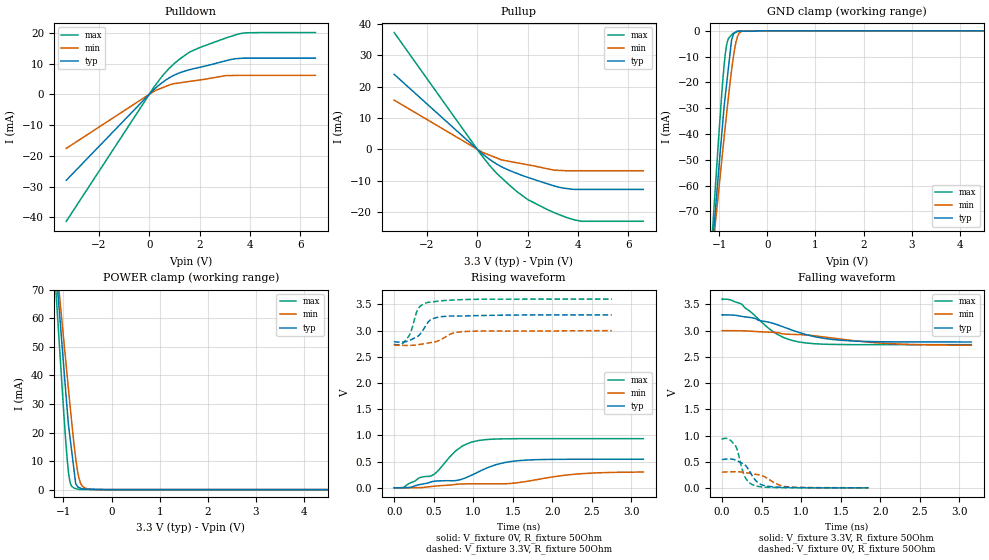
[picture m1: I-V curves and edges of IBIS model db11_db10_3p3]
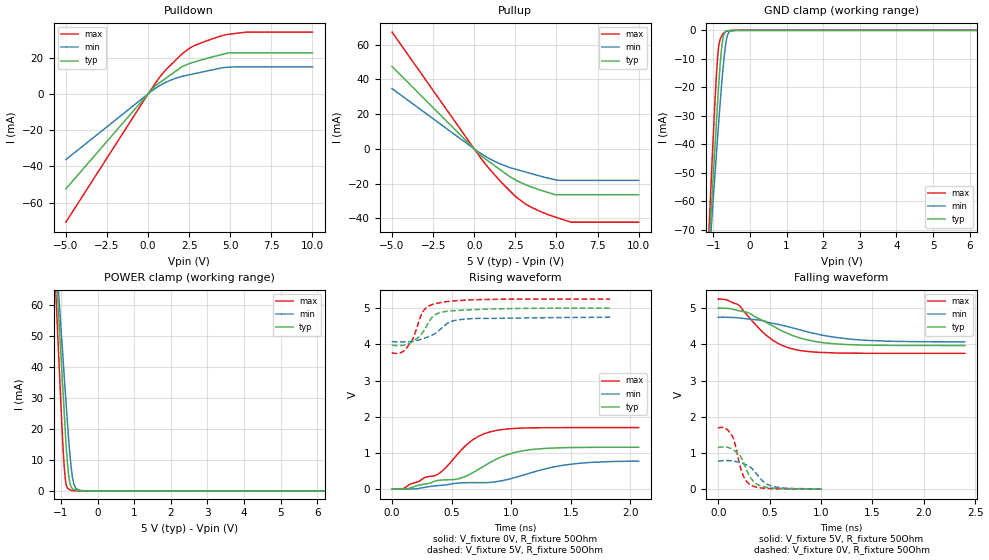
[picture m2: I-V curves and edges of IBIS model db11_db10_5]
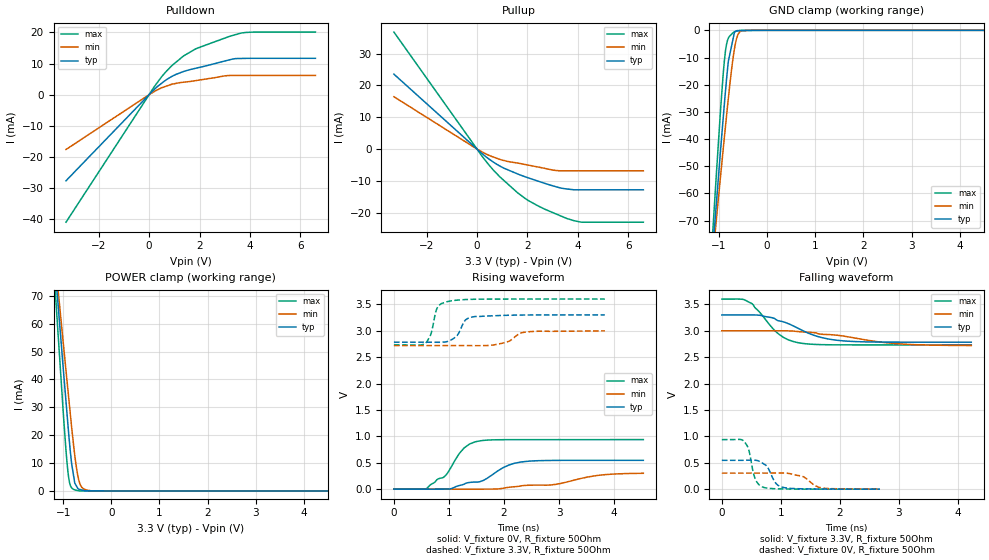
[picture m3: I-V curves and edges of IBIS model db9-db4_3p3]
|Texas Instruments Incorporated
| 2.7V-5.25V Digital, 5V Analog, 12 Bit, 3MSPS, Parallel ADC with Ref
| Marketing part#   Digital Voltage Range   Package-type   #pins
| ADS7882IPFBR   2.7V-5.25V   TQFP   48
| ADS7882IPFBT   2.7V-5.25V   TQFP   48
[IBIS Ver]   3.2
[File name]   ads7882.ibs
|SIMDE Ver   V2.2 - 201009 - RHL4 - Build 424
[File Rev]   1.1
[Date]   4/15/2011
[Source]
| Texas Instruments Incorporated.
| Analog-eLab Design Center, HPA
| 12500 TI Blvd
| Dallas, TX -75243
| e-mail: elab_ibis@list.ti.com
| -Model generated from simulations in SPECTRE
[Notes]   Revision History:
| Rev 1.0: 4/8/2011
| - Initial version of the model
| - Model generated from simulations in SPECTRE
| - Model matched to SPICE simulation
| - C_comp although listed in numerical order of value are
|   obtained from varying PVT conditions. For PVT conditions for
|   each specific value refer the buffer description under
|   respective [Model]. IBIS model user is responsible for using
|   appropriate C_comp to simulate for Signal Integrity.
| - Model names with a trailing _3p3 contains the model for
|   3.3V [3.0V and 3.6V].Model names with a trailing _5 contains
|   the model for 5.0V [4.75V and 5.25V].
|   Rev 1.1: 4/15/2011
| - Updated the IBIS model with LC tank C_Comp
[Disclaimer]
| This model is designed as an aid for customers of Texas Instruments.
| TI and its licensors and suppliers make no warranties, either expressed
| or implied, with respect to this  model, including the warranties of
| merchantability or fitness for a particular purpose. The model is
| provided solely on an "as is" basis. The entire risk as to its quality
| and performance is with the customer.
[Copyright]
 (C) Copyright 2011 Texas Instruments Incorporated.All rights reserved.
|   ADS7882
[Component]   ADS7882
[Manufacturer]   TI
[Package]   |48 TQFP - PFB package
|   typ   min   max
R_pkg   0.096154   0.08201   0.10924
L_pkg   2.99219nH   2.49975nH   3.83153nH
C_pkg   0.482595pF   0.40017pF   0.58535pF
[Pin]  signal_name   model_name   R_pin   L_pin   C_pin
1   REFIN   TERM   0.10156   3.67689nH  0.57752pF
2   REFOUT   TERM   0.09278   2.95431nH  0.50865pF
3   NC   NC   0.08775   2.81037nH  0.48710pF
4   +VA   POWER   0.08458   2.75529nH  0.48008pF
5   AGND   GND   0.08266   2.53910nH  0.43335pF
6   IN+   TERM   0.08227   2.50412nH  0.40022pF
7   -IN   TERM   0.08210   2.49975nH  0.40017pF
8   AGND   GND   0.08205   2.52717nH  0.43280pF
9   +VA   POWER   0.08351   2.73719nH  0.47819pF
10   +VA   POWER   0.08625   2.78317nH  0.48546pF
11   AGND   GND   0.09077   2.91560nH  0.51015pF
12   AGND   GND   0.04966   3.05669nH  0.63306pF
13   +VA   POWER   0.11087   3.87375nH  0.58548pF
14   AGND   GND   0.10407   3.18780nH  0.51804pF
15   AGND   GND   0.10062   3.07419nH  0.49891pF
16   DB11   DB   0.09878   3.04135nH  0.49726pF
17   DB10   DB   0.09794   2.84794nH  0.45076pF
18   DB9   DB9-DB3   0.09833   2.82757nH  0.41819pF
19   DB8   DB9-DB3   0.09865   2.83183nH  0.41907pF
20   DB7   DB9-DB3   0.09892   2.86570nH  0.45238pF
21   DB6   DB9-DB3   0.10045   3.07454nH  0.49862pF
22   DB5   DB9-DB3   0.10298   3.12010nH  0.50228pF
23   DB4   DB9-DB3   0.10708   3.24374nH  0.52526pF
24   +VBD   POWER   0.11463   3.93871nH  0.59461pF
25   BDGND   GND   0.09909   3.63469nH  0.57452pF
26   DB3   DB9-DB3   0.09081   2.92111nH  0.50606pF
27   DB2   DB   0.08620   2.78437nH  0.48513pF
28   DB1   DB   0.08347   2.73669nH  0.47871pF
29   DB0   DB0   0.08201   2.52810nH  0.43255pF
30   NC   NC   0.08207   2.50072nH  0.39994pF
31   NC   NC   0.08234   2.50365nH  0.40065pF
32   NC   NC   0.08284   2.54077nH  0.43406pF
33   NC   NC   0.08487   2.76069nH  0.47992pF
34   +VBD   POWER   0.08812   2.81537nH  0.48776pF
35   BDGND   GND   0.09307   2.95530nH  0.51266pF
36   BUSY   BUSY   0.10188   3.67198nH  0.58535pF
37   _A_PWD   INPUT   0.10924   3.83153nH  0.58324pF
38   _PWD/_RST   INPUT   0.10264   3.15016nH  0.51710pF
39   BYTE   BYTE   0.09952   3.04261nH  0.49838pF
40   _CONVST   INPUT   0.09803   3.01798nH  0.49502pF
41   _RD   INPUT   0.09757   2.83036nH  0.44993pF
42   _CS   INPUT   0.09834   2.81763nH  0.41784pF
43   +VA   POWER   0.09896   2.82837nH  0.41883pF
44   AGND   GND   0.09951   2.86775nH  0.45275pF
45   AGND   GND   0.10137   3.08409nH  0.49933pF
46   +VA   POWER   0.10424   3.13488nH  0.50621pF
47   REFM   GND   0.05396   2.70861nH  0.58111pF
48   REFM   GND   0.10969   3.82962nH  0.59256pF
|   Model Selectors
[Model Selector] DB
db11_db10_3p3   3.3V digital 3-state output
db11_db10_5   5.0V digital 3-state output
[Model Selector] DB9-DB3
db9-db4_3p3   3.3V digital 3-state output
db9-db4_5   5.0V digital 3-state output
[Model Selector] DB0
db0_par_3p3   3.3V digital 3-state output
db0_par_5   5.0V digital 3-state output
[Model Selector] BUSY
busy_3p3   3.3V digital output
busy_5   5.0V digital output
[Model Selector] INPUT
input_3p3   3.3V digital input
input_5   5.0V digital input
[Model Selector] BYTE
byte_3p3   3.3V digital input
byte_5   5.0V digital input
[Model Selector] TERM
term_3-3V   3.3V nominal termination
term_5-0V   5.0V nominal termination
[Model]  term_3-3V
Model_type Terminator
C_comp   1.0e-20F  1.0e-20F  1.0e-20F
|   typ   min   max
[Voltage Range]   3.3V   3.0V   3.6V
[POWER Clamp Reference]   3.3V   3.0V   3.6V
[GND Clamp Reference]   0V   0V   0V
|Ambient Temperature   25   85   -40
|Junction Temperature
[Temperature Range]   25   85   -40
[Model]  term_5-0V
Model_type Terminator
C_comp   1.0e-20F  1.0e-20F  1.0e-20F
|   typ   min   max
[Voltage Range]   5.0V   4.75V   5.25V
[POWER Clamp Reference]   5.0V   4.75V   5.25V
[GND Clamp Reference]   0V   0V   0V
|Ambient Temperature   25   85   -40
|Junction Temperature
[Temperature Range]   25   85   -40
| Models and submodels in the file (14): db11_db10_3p3 (3-state), db11_db10_5 (3-state), db9-db4_3p3 (3-state), db9-db4_5 (3-state), db0_par_3p3 (3-state), db0_par_5 (3-state), busy_3p3 (Output), busy_5 (Output), input_3p3 (Input), input_5 (Input), byte_3p3 (Input), byte_5 (Input), term_3-3V (Terminator), term_5-0V (Terminator)
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|   db11_db10_3p3 Model
[Model]   db11_db10_3p3
Model_type   3-state
Polarity   Non-Inverting
Enable   Active-Low
Vmeas = 1.65
Vref = 1.65
Cref = 20pF
Rref = 50
|   typ   min   max
|   (nom PVT)   (Fast PVT)   (slow PVT)
|C_comp from frequency sweep method (F=1.5MHz)
|Average
C_comp   1.207e-12   1.083e-12   1.350e-12
|ON state : BUFFER OUTPUT TURNED HIGH
|C_comp   1.164e-12   1.043e-12   1.312e-12
|OFF state: BUFFER IN HIGH IMPEDANCE
|C_comp   1.251e-12   1.124e-12   1.388e-12
|C_comp from LC tank measurement(L=1nH)
|Resonant Frequency(Hz)   5.950e+09   6.040e+09   5.790e+09
|C_comp   7.162e-13   6.950e-13   7.564e-13
|ON state : BUFFER OUTPUT TURNED HIGH
|Resonant Frequency(Hz)   5.950e+09   6.040e+09   5.790e+09
|C_comp   7.162e-13   6.950e-13   7.564e-13
|OFF state: BUFFER IN HIGH IMPEDANCE
|Resonant Frequency   5.980e+09   6.040e+09   5.270e+09
|C_comp   7.091e-13   6.950e-13   9.130e-13
| Where nom  PVT is Nominal Process,  3.3V,  25C
|   Fast PVT is Strong Process,   3.6V,  -40C
|   Slow PVT is Weak Process,   3V,  85C
[Voltage Range]   3.3   3   3.6
|Ambient Temperature   25   85   -40
|Junction Temperature
[Temperature Range]   25   85   -40
[Pullup Reference]   3.3   3   3.6
[Pulldown Reference]   0   0   0
[Power Clamp Reference]   3.3   3   3.6
[GND Clamp Reference]   0   0   0
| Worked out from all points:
|   slope of the pulldown table from 0 to 0.495 V, typ, clamps not added: 134 ohm
|   slope of the pullup table from 0 to 0.495 V, typ, clamps not added: 152 ohm
|   GND clamp passes 1 mA (typ) near -0.69 V on its own axis
|   POWER clamp passes 1 mA (typ) near -0.70 V on its own axis
|   falling waveform, V_fixture 3.3V, R_fixture 50Ohm: 20-80 % time 702ps typ, 1.13ns min, 431ps max; typ from 3.3 V to 2.78 V
|   rising waveform, V_fixture 0V, R_fixture 50Ohm: 20-80 % time 821ps typ, 1.41ns min, 506ps max; typ from 0 V to 0.545 V
|   rising waveform, V_fixture 3.3V, R_fixture 50Ohm: 20-80 % time 161ps typ, 254ps min, 118ps max; typ from 2.78 V to 3.3 V
|   falling waveform, V_fixture 0V, R_fixture 50Ohm: 20-80 % time 154ps typ, 224ps min, 112ps max; typ from 0.546 V to 0.001 V
[Pulldown]
|   Voltage   I(typ)   I(min)   I(max)
-3.3V     -27.98mA   -17.6mA    -41.31mA
165.6mV   1.385mA    845.6uA    2.114mA
489.6mV   3.669mA    2.022mA    5.683mA
795.6mV   5.364mA    3.005mA    8.487mA
1.256V    7.123mA    3.771mA    11.75mA
1.62V     8.032mA    4.204mA    13.79mA
2.023V    8.799mA    4.669mA    15.25mA
3.024V    10.86mA    6.055mA    18.24mA
3.561V    11.65mA    6.146mA    19.63mA
3.863V    11.74mA    6.146mA    19.99mA
4.392V    11.74mA    6.146mA    20.06mA
6.6V      11.74mA    6.146mA    20.06mA
[GND Clamp]
|   Voltage   I(typ)   I(min)   I(max)
-3.3V     -576.2mA   -485.3mA   -699.8mA
-1.145V   -84.01mA   -86.27mA   -78.64mA
-1.116V   -77.47mA   -80.95mA   -70.35mA
-1.015V   -54.79mA   -62.53mA   -42.05mA
-943.2mV  -38.9mA    -49.37mA   -23.1mA
-874.8mV  -25.19mA   -37.02mA   -8.97mA
-831.6mV  -18.02mA   -29.41mA   -4.204mA
-745.8mV  -3.777mA   -15.46mA   -1.608mA
-640.2mV  -175.5uA   -3.504mA   -449.1uA
-585mV    -160.3uA   -878.4uA   -96.21uA
-441mV    -120.6uA   -12.32uA   -49.56uA
6.6V      0A         0A         0A
[Pullup]
|   Voltage   I(typ)   I(min)   I(max)
-3.3V     23.88mA    15.66mA    37.21mA
133.2mV   -958.5uA   -613uA     -1.531mA
489.6mV   -3.219mA   -1.877mA   -5.159mA
795.6mV   -4.826mA   -2.854mA   -7.853mA
963mV     -5.573mA   -3.388mA   -9.095mA
1.562V    -7.652mA   -4.286mA   -13.42mA
2.023V    -9.002mA   -4.966mA   -16.1mA
2.79V     -11.02mA   -6.217mA   -19.25mA
3.251V    -12.11mA   -6.733mA   -20.84mA
3.863V    -12.8mA    -6.845mA   -22.52mA
4.14V     -12.8mA    -6.845mA   -22.97mA
6.6V      -12.8mA    -6.845mA   -22.97mA
[POWER Clamp]
|   Voltage   I(typ)   I(min)   I(max)
-3.3V     535.6mA    459.6mA    634.1mA
-1.494V   149.6mA    140.6mA    158mA
-1.066V   58.37mA    65.16mA    45.83mA
-954mV    34.64mA    45.45mA    17.39mA
-896.4mV  22.77mA    35.3mA     6.276mA
-849.6mV  16.36mA    27.25mA    1.888mA
-774mV    6.003mA    15.03mA    480.7uA
-742.5mV  1.995mA    10.65mA    356.5uA
-702mV    960.8uA    6.073mA    196.8uA
-642mV    473.3uA    2.131mA    25.18uA
-441mV    169.7uA    94.34uA    10.88uA
6.6V      0A         0A         0A
[Ramp]
R_load = 50
|   typ   min   max
dV/dt_r   0.32766/8.22315e-10   0.182251/1.42229e-09   0.563074/5.05939e-10
dV/dt_f   0.310142/7.04688e-10   0.168714/1.14884e-09   0.520813/4.31957e-10
[Falling Waveform]
V_fixture = 3.3V
V_fixture_min = 3V
V_fixture_max = 3.6V
R_fixture = 50Ohm
|   Time   V(typ)   V(min)   V(max)
0s        3.3V       3V         3.6V
101.4ps   3.299V     3.001V     3.59V
249.2ps   3.272V     2.997V     3.503V
629.5ps   3.147V     2.969V     2.998V
776ps     3.071V     2.939V     2.871V
966.7ps   2.969V     2.925V     2.786V
1.296ns   2.852V     2.879V     2.742V
1.596ns   2.808V     2.822V     2.735V
2.254ns   2.786V     2.744V     2.733V
3.154ns   2.784V     2.722V     2.733V
[Rising Waveform]
V_fixture = 0V
V_fixture_min = 0V
V_fixture_max = 0V
R_fixture = 50Ohm
|   Time   V(typ)   V(min)   V(max)
0s        1.565nV    6.201nV    1.48nV
119.2ps   1.329mV    -140.3uV   11.04mV
317.5ps   60.29mV    3.418mV    190.2mV
484.1ps   119.7mV    27mV       238.9mV
776ps     138.5mV    64.82mV    702mV
1.066ns   304.4mV    76.04mV    902.4mV
1.296ns   444.9mV    76.28mV    931.1mV
1.596ns   521.2mV    104.6mV    937.4mV
2.354ns   544.9mV    267.8mV    937.7mV
3.154ns   545.3mV    301mV      937.9mV
[Rising Waveform]
V_fixture = 3.3V
V_fixture_min = 3V
V_fixture_max = 3.6V
R_fixture = 50Ohm
|   Time   V(typ)   V(min)   V(max)
0s        2.783V     2.719V     2.732V
101.4ps   2.78V      2.717V     2.749V
182.3ps   2.806V     2.716V     2.887V
215.1ps   2.828V     2.718V     2.993V
299.8ps   2.893V     2.73V      3.408V
431.8ps   3.166V     2.763V     3.54V
570.8ps   3.259V     2.813V     3.565V
752.2ps   3.277V     2.955V     3.583V
871ps     3.279V     2.979V     3.591V
2.754ns   3.299V     2.999V     3.6V
[Falling Waveform]
V_fixture = 0V
V_fixture_min = 0V
V_fixture_max = 0V
R_fixture = 50Ohm
|   Time   V(typ)   V(min)   V(max)
0s        546.1mV    303.8mV    938.4mV
86.69ps   552.5mV    306.4mV    931.7mV
163.7ps   533.8mV    308.7mV    815.3mV
190.6ps   516.4mV    307.9mV    726.7mV
283.3ps   446.9mV    296.7mV    226.2mV
334.7ps   350.7mV    282.3mV    114.6mV
407.8ps   171.3mV    262.6mV    46.38mV
508.1ps   55.61mV    232.7mV    17.77mV
795.9ps   9.999mV    27.3mV     3.728mV
1.854ns   1.112mV    1.732mV    947uV
|   db11_db10_5 Model
[Model]   db11_db10_5
Model_type   3-state
Polarity   Non-Inverting
Enable   Active-Low
Vmeas = 2.5
Vref = 2.5
Cref = 20pF
Rref = 50
|   typ   min   max
|   (nom PVT)   (Fast PVT)   (slow PVT)
|C_comp from frequency sweep method (F=1.5MHz)
|Average
C_comp   1.103e-12   1.013e-12   1.196e-12
|ON state : BUFFER OUTPUT TURNED HIGH
|C_comp   1.072e-12   9.914e-13   1.154e-12
|OFF state: BUFFER IN HIGH IMPEDANCE
|C_comp   1.135e-12   1.036e-12   1.237e-12
|C_comp from LC tank measurement(L=1nH)
|Resonant Frequency(Hz)   6.030e+09   6.110e+09   5.860e+09
|C_comp   6.973e-13   6.792e-13   7.384e-13
|ON state : BUFFER OUTPUT TURNED HIGH
|Resonant Frequency(Hz)   6.030e+09   6.110e+09   5.860e+09
|C_comp   6.973e-13   6.792e-13   7.384e-13
|OFF state: BUFFER IN HIGH IMPEDANCE
|Resonant Frequency   6.000e+09   6.070e+09   5.330e+09
|C_comp   7.043e-13   6.882e-13   8.925e-13
| Where nom  PVT is Nominal Process,  5V,  25C
|   Fast PVT is Strong Process,   5.25V,  -40C
|   Slow PVT is Weak Process,   4.75V,  85C
[Voltage Range]   5   4.75   5.25
|Ambient Temperature   25   85   -40
|Junction Temperature
[Temperature Range]   25   85   -40
[Pullup Reference]   5   4.75   5.25
[Pulldown Reference]   0   0   0
[Power Clamp Reference]   5   4.75   5.25
[GND Clamp Reference]   0   0   0
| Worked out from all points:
|   slope of the pulldown table from 0 to 0.75 V, typ, clamps not added: 115 ohm
|   slope of the pullup table from 0 to 0.75 V, typ, clamps not added: 119 ohm
|   GND clamp passes 1 mA (typ) near -0.69 V on its own axis
|   POWER clamp passes 1 mA (typ) near -0.70 V on its own axis
|   falling waveform, V_fixture 5V, R_fixture 50Ohm: 20-80 % time 457ps typ, 632ps min, 328ps max; typ from 5 V to 3.97 V
|   rising waveform, V_fixture 0V, R_fixture 50Ohm: 20-80 % time 572ps typ, 852ps min, 380ps max; typ from 0 V to 1.16 V
|   rising waveform, V_fixture 5V, R_fixture 50Ohm: 20-80 % time 138ps typ, 182ps min, 112ps max; typ from 3.97 V to 5 V
|   falling waveform, V_fixture 0V, R_fixture 50Ohm: 20-80 % time 125ps typ, 158ps min, 96.5ps max; typ from 1.16 V to 0.004 V
[Pulldown]
|   Voltage   I(typ)   I(min)   I(max)
-5V       -52.47mA   -36.3mA    -70.88mA
5mV       107.6uA    73.76uA    142uA
485mV     4.823mA    3.296mA    6.403mA
708.7mV   6.272mA    4.614mA    9.321mA
1.377V    10.6mA     7.65mA     16mA
2.05V     14.95mA    9.707mA    21.97mA
2.494V    16.67mA    10.57mA    25.11mA
3.16V     18.58mA    11.86mA    27.96mA
4.756V    22.38mA    14.69mA    32.83mA
6.011V    22.7mA     14.91mA    34.18mA
10V       22.7mA     14.91mA    34.18mA
[GND Clamp]
|   Voltage   I(typ)   I(min)   I(max)
-5V       -967.7mA   -802.9mA   -1.193A
-1.306V   -120mA     -115.5mA   -124mA
-1.09V    -71.21mA   -75.88mA   -62.73mA
-1.024V   -56.7mA    -63.75mA   -43.95mA
-918.7mV  -33.7mA    -44.52mA   -17.02mA
-866.2mV  -22.21mA   -35.23mA   -7.498mA
-808.5mV  -11.66mA   -25.26mA   -2.927mA
-760mV    -5.001mA   -17.33mA   -1.792mA
-645mV    -192.6uA   -3.734mA   -341uA
-565.3mV  -124.5uA   -479.8uA   -127uA
-384.7mV  -297.3nA   -2.013uA   -3.392uA
10V       0A         0A         0A
[Pullup]
|   Voltage   I(typ)   I(min)   I(max)
-5V       47.49mA    34.75mA    67.31mA
504mV     -4.587mA   -3.237mA   -6.658mA
1.377V    -10.63mA   -7.806mA   -16.4mA
2.05V     -15.28mA   -10.36mA   -23.09mA
2.557V    -18.11mA   -11.82mA   -27.84mA
3.16V     -20.77mA   -13.42mA   -32.01mA
3.607V    -22.39mA   -14.6mA    -34.28mA
4.945V    -26.42mA   -17.8mA    -39.31mA
5.891V    -26.42mA   -18.16mA   -42.25mA
10V       -26.42mA   -18.16mA   -42.25mA
[POWER Clamp]
|   Voltage   I(typ)   I(min)   I(max)
-5V       900mA      760.5mA    1.084A
-1.306V   109.2mA    107.1mA    108.3mA
-1.09V    63.13mA    69.07mA    51.76mA
-1.008V   46.08mA    54.65mA    30.31mA
-934.5mV  30.79mA    41.73mA    12.76mA
-882mV    19.87mA    32.49mA    4.239mA
-785mV    4.745mA    16.41mA    605uA
-714mV    1.238mA    7.241mA    157.2uA
-646mV    418.6uA    2.22mA     56.96uA
-593.8mV  316.7uA    932.4uA    2.329uA
-332.5mV  355.7nA    4.212uA    786nA
10V       0A         0A         0A
[Ramp]
R_load = 50
|   typ   min   max
dV/dt_r   0.694763/5.72602e-10   0.468296/8.5622e-10   1.01977/3.80376e-10
dV/dt_f   0.61811/4.56691e-10   0.408104/6.31353e-10   0.898003/3.28008e-10
[Falling Waveform]
V_fixture = 5V
V_fixture_min = 4.75V
V_fixture_max = 5.25V
R_fixture = 50Ohm
|   Time   V(typ)   V(min)   V(max)
0s        5V         4.75V      5.25V
77.83ps   4.996V     4.75V      5.236V
189.8ps   4.937V     4.738V     5.104V
302.8ps   4.862V     4.699V     4.74V
483.5ps   4.584V     4.613V     4.216V
627.5ps   4.366V     4.527V     3.967V
771.5ps   4.2V       4.422V     3.846V
1.017ns   4.05V      4.254V     3.778V
1.351ns   3.988V     4.13V      3.757V
2.4ns     3.97V      4.07V      3.753V
[Rising Waveform]
V_fixture = 0V
V_fixture_min = 0V
V_fixture_max = 0V
R_fixture = 50Ohm
|   Time   V(typ)   V(min)   V(max)
0s        2.197nV    6.551nV    2.052nV
90.21ps   3.083mV    -5.611uV   11.18mV
279.9ps   141.1mV    50.54mV    325.7mV
377.5ps   232.9mV    92.98mV    397mV
627.5ps   367.3mV    176.6mV    1.23V
819.5ps   728.6mV    183.9mV    1.579V
1.017ns   999.7mV    306mV      1.673V
1.209ns   1.105V     492.7mV    1.694V
1.543ns   1.15V      703.2mV    1.699V
2.071ns   1.157V     774.7mV    1.699V
[Rising Waveform]
V_fixture = 5V
V_fixture_min = 4.75V
V_fixture_max = 5.25V
R_fixture = 50Ohm
|   Time   V(typ)   V(min)   V(max)
0s        3.969V     4.068V     3.753V
67.08ps   3.965V     4.066V     3.761V
122.2ps   3.997V     4.068V     3.899V
177.7ps   4.087V     4.085V     4.171V
263ps     4.352V     4.158V     4.923V
336.2ps   4.744V     4.253V     5.099V
386.9ps   4.858V     4.361V     5.138V
482.4ps   4.924V     4.611V     5.189V
607.7ps   4.946V     4.696V     5.218V
1.831ns   4.999V     4.748V     5.25V
[Falling Waveform]
V_fixture = 0V
V_fixture_min = 0V
V_fixture_max = 0V
R_fixture = 50Ohm
|   Time   V(typ)   V(min)   V(max)
0s        1.158V     782.7mV    1.7V
67.08ps   1.165V     788.4mV    1.688V
132.7ps   1.111V     783.1mV    1.489V
159.9ps   1.06V      772.2mV    1.293V
206.2ps   951.6mV    741mV      716.9mV
246.6ps   737.8mV    700.8mV    354.6mV
319ps     300.6mV    594.1mV    109.5mV
386.9ps   121.6mV    374.3mV    46.93mV
507.8ps   37.05mV    96mV       16.19mV
1.011ns   3.964mV    7.67mV     537.8uV
|   db9-db4_3p3 Model
[Model]   db9-db4_3p3
Model_type   3-state
Polarity   Non-Inverting
Enable   Active-Low
Vmeas = 1.65
Vref = 1.65
Cref = 20pF
Rref = 50
|   typ   min   max
|   (nom PVT)   (Fast PVT)   (slow PVT)
|C_comp from frequency sweep method (F=1.5MHz)
|Average
C_comp   1.231e-12   1.113e-12   1.343e-12
|ON state : BUFFER OUTPUT TURNED HIGH
|C_comp   1.186e-12   1.072e-12   1.305e-12
|OFF state: BUFFER IN HIGH IMPEDANCE
|C_comp   1.275e-12   1.154e-12   1.381e-12
|C_comp from LC tank measurement(L=1nH)
|Resonant Frequency(Hz)   5.950e+09   6.030e+09   5.790e+09
|C_comp   7.162e-13   6.973e-13   7.564e-13
|ON state : BUFFER OUTPUT TURNED HIGH
|Resonant Frequency(Hz)   5.950e+09   6.030e+09   5.790e+09
|C_comp   7.162e-13   6.973e-13   7.564e-13
|OFF state: BUFFER IN HIGH IMPEDANCE
|Resonant Frequency   5.980e+09   6.030e+09   5.270e+09
|C_comp   7.091e-13   6.973e-13   9.130e-13
| Where nom  PVT is Nominal Process,  3.3V,  25C
|   Fast PVT is Strong Process,   3.6V,  -40C
|   Slow PVT is Weak Process,   3V,  85C
[Voltage Range]   3.3   3   3.6
|Ambient Temperature   25   85   -40
|Junction Temperature
[Temperature Range]   25   85   -40
[Pullup Reference]   3.3   3   3.6
[Pulldown Reference]   0   0   0
[Power Clamp Reference]   3.3   3   3.6
[GND Clamp Reference]   0   0   0
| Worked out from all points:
|   slope of the pulldown table from 0 to 0.495 V, typ, clamps not added: 136 ohm
|   slope of the pullup table from 0 to 0.495 V, typ, clamps not added: 153 ohm
|   GND clamp passes 1 mA (typ) near -0.68 V on its own axis
|   POWER clamp passes 1 mA (typ) near -0.70 V on its own axis
|   falling waveform, V_fixture 3.3V, R_fixture 50Ohm: 20-80 % time 701ps typ, 1.13ns min, 432ps max; typ from 3.3 V to 2.78 V
|   rising waveform, V_fixture 0V, R_fixture 50Ohm: 20-80 % time 745ps typ, 1.27ns min, 457ps max; typ from 0 V to 0.546 V
|   rising waveform, V_fixture 3.3V, R_fixture 50Ohm: 20-80 % time 170ps typ, 267ps min, 123ps max; typ from 2.78 V to 3.3 V
|   falling waveform, V_fixture 0V, R_fixture 50Ohm: 20-80 % time 156ps typ, 230ps min, 114ps max; typ from 0.546 V to 0 V
[Pulldown]
|   Voltage   I(typ)   I(min)   I(max)
-3.3V     -27.67mA   -17.62mA   -40.96mA
202.8mV   1.678mA    1.001mA    2.556mA
638.4mV   4.547mA    2.61mA     7.114mA
908.4mV   5.876mA    3.361mA    9.385mA
1.369V    7.443mA    3.996mA    12.44mA
1.916V    8.597mA    4.592mA    14.92mA
3.018V    10.84mA    6.049mA    18.21mA
3.432V    11.58mA    6.178mA    19.28mA
3.655V    11.62mA    6.178mA    19.79mA
4.138V    11.67mA    6.178mA    20.09mA
6.6V      11.67mA    6.178mA    20.09mA
[GND Clamp]
|   Voltage   I(typ)   I(min)   I(max)
-3.3V     -576.2mA   -485.5mA   -699.8mA
-1.439V   -150.4mA   -140.3mA   -162.4mA
-1.061V   -65.15mA   -70.79mA   -54.73mA
-970.8mV  -44.85mA   -54.32mA   -30.09mA
-913.2mV  -32.43mA   -43.85mA   -16.17mA
-862.8mV  -21.92mA   -34.93mA   -7.26mA
-805.2mV  -11.37mA   -24.96mA   -2.865mA
-676.5mV  -531.9uA   -6.573mA   -557.3uA
-623.7mV  -107uA     -2.45mA    -235.5uA
-546mV    -91.27uA   -288.4uA   -27.28uA
-369mV    -55.4uA    -756.4nA   0A
6.6V      0A         0A         0A
[Pullup]
|   Voltage   I(typ)   I(min)   I(max)
-3.3V     23.54mA    16.46mA    36.76mA
202.8mV   -1.439mA   -911.4uA   -2.28mA
638.4mV   -4.038mA   -2.462mA   -6.518mA
901.2mV   -5.306mA   -3.232mA   -8.691mA
1.6V      -7.773mA   -4.37mA    -13.66mA
2.053V    -9.09mA    -5.062mA   -16.25mA
2.467V    -10.19mA   -5.705mA   -18.04mA
3.156V    -11.88mA   -6.741mA   -20.45mA
3.846V    -12.79mA   -6.823mA   -22.49mA
4.138V    -12.8mA    -6.823mA   -22.96mA
6.6V      -12.8mA    -6.823mA   -22.96mA
[POWER Clamp]
|   Voltage   I(typ)   I(min)   I(max)
-3.3V     535.6mA    459.6mA    634.1mA
-1.575V   166.9mA    154.8mA    179.5mA
-999.6mV  44.28mA    53.44mA    28.58mA
-942mV    32.27mA    43.29mA    14.7mA
-898.8mV  23.28mA    35.82mA    6.629mA
-848.4mV  13.75mA    27.11mA    1.831mA
-794.4mV  6.637mA    18.16mA    645.2uA
-759mV    2.841mA    12.84mA    402.8uA
-705mV    1.181mA    6.362mA    154.2uA
-648mV    509.2uA    2.376mA    25.09uA
-426mV    53.28uA    66.02uA    0A
6.6V      0A         0A         0A
[Ramp]
R_load = 50
|   typ   min   max
dV/dt_r   0.327661/7.4475e-10   0.181829/1.28267e-09   0.563067/4.5683e-10
dV/dt_f   0.310179/7.01037e-10   0.168589/1.13797e-09   0.520866/4.32355e-10
[Falling Waveform]
V_fixture = 3.3V
V_fixture_min = 3V
V_fixture_max = 3.6V
R_fixture = 50Ohm
|   Time   V(typ)   V(min)   V(max)
0s        3.3V       3V         3.6V
348.4ps   3.3V       3V         3.597V
503.4ps   3.3V       3V         3.52V
939.1ps   3.199V     3V         2.962V
1.114ns   3.141V     2.999V     2.835V
1.278ns   3.055V     2.986V     2.778V
1.687ns   2.873V     2.935V     2.737V
2.087ns   2.806V     2.895V     2.733V
2.943ns   2.784V     2.758V     2.732V
4.232ns   2.783V     2.72V      2.732V
[Rising Waveform]
V_fixture = 0V
V_fixture_min = 0V
V_fixture_max = 0V
R_fixture = 50Ohm
|   Time   V(typ)   V(min)   V(max)
0s        1.565nV    6.201nV    1.48nV
594.8ps   289.6uV    18.11uV    13.88mV
939.1ps   1.194mV    28.59uV    259.2mV
1.278ns   95.66mV    38.9uV     783.3mV
1.478ns   133.4mV    44.99uV    897mV
2.087ns   456.2mV    35.24mV    937.6mV
2.387ns   524.2mV    70.96mV    937.7mV
2.943ns   544.6mV    91.44mV    937.8mV
3.832ns   546mV      274.3mV    938.1mV
4.532ns   546.1mV    300.6mV    938.3mV
[Rising Waveform]
V_fixture = 3.3V
V_fixture_min = 3V
V_fixture_max = 3.6V
R_fixture = 50Ohm
|   Time   V(typ)   V(min)   V(max)
0s        2.783V     2.719V     2.732V
576.7ps   2.783V     2.719V     2.767V
675.3ps   2.782V     2.719V     2.947V
782.3ps   2.782V     2.719V     3.424V
977.5ps   2.798V     2.719V     3.553V
1.301ns   3.206V     2.718V     3.591V
1.44ns    3.263V     2.718V     3.595V
2.012ns   3.291V     2.775V     3.6V
2.376ns   3.298V     2.973V     3.6V
3.832ns   3.3V       2.998V     3.6V
[Falling Waveform]
V_fixture = 0V
V_fixture_min = 0V
V_fixture_max = 0V
R_fixture = 50Ohm
|   Time   V(typ)   V(min)   V(max)
0s        546.1mV    303.8mV    938.4mV
373ps     547mV      303.9mV    912.1mV
459.2ps   549mV      303.9mV    736.6mV
557.6ps   549mV      303.9mV    217.8mV
707.3ps   480mV      304.5mV    34.23mV
918ps     108.4mV    306.6mV    7.485mV
1.041ns   33.71mV    306.1mV    3.952mV
1.359ns   7.013mV    245.9mV    800.6uV
1.696ns   2.566mV    23.61mV    274.6uV
2.679ns   84.4uV     1.969mV    3.682uV
